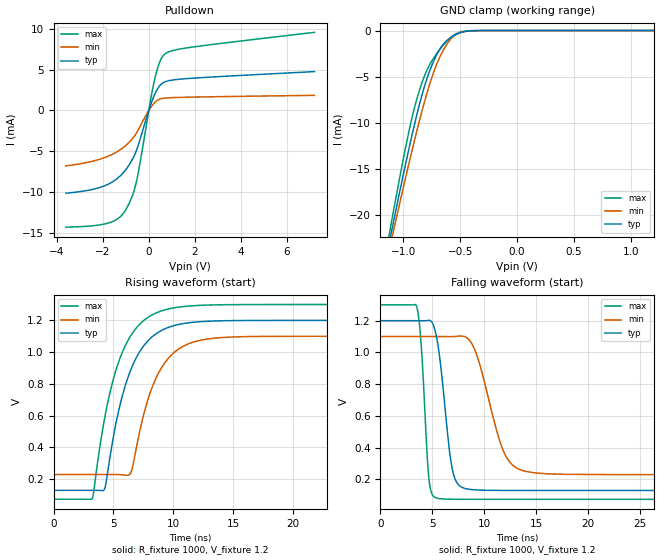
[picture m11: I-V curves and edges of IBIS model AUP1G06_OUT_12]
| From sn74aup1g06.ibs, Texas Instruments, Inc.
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[Model]   AUP1G06_OUT_12
Model_type  Open_drain
Enable   Active-Low
Vref =   1.2
Rref =   1E6
Cref =   30p
Vmeas =   0.6
| variable   typ   min   max
C_comp   1.72pF   1.50pF   1.95pF
| C_pulldown   2.12pF   1.69pF   2.59pF
| C_tri-state   1.72pF   1.50pF   1.95pF
[Temperature Range]   40   100   -40
| Ambient temperature   25   85   -40
[Voltage range]   1.2   1.1   1.3
[Pullup Reference]   1.2   1.2   1.2
[POWER Clamp Reference]   1.2   1.2   1.2
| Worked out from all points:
|   slope of the pulldown table from 0 to 0.18 V, typ, clamps not added: 125 ohm
|   GND clamp passes 1 mA (typ) near -0.61 V on its own axis
|   rising waveform, R_fixture 1000, V_fixture 1.2: 20-80 % time 2.34ns typ, 2.3ns min, 2.38ns max; typ from 0.129 V to 1.2 V
|   falling waveform, R_fixture 1000, V_fixture 1.2: 20-80 % time 1.05ns typ, 2.14ns min, 612ps max; typ from 1.2 V to 0.129 V
[GND Clamp]
| AUP1G06_OUT_12
|   Voltage   I(typ)   I(min)   I(max)
-3.6V     -193.5mA   -179.7mA   -210.2mA
-1.12V    -22.9mA    -23.71mA   -21.96mA
-1.1V     -21.68mA   -22.59mA   -20.6mA
-1.08V    -20.46mA   -21.47mA   -19.24mA
-935mV    -12.04mA   -13.67mA   -10.14mA
-835mV    -6.999mA   -8.739mA   -5.664mA
-765mV    -4.303mA   -5.73mA    -3.651mA
-690mV    -2.262mA   -3.202mA   -2.243mA
-615mV    -1.069mA   -1.462mA   -1.136mA
-550mV    -509uA     -564.1uA   -463.6uA
-340mV    -5.773uA   -7.668uA   -1.491uA
1.2V      118.1pA    564.4pA    21.05pA
[Pulldown]
| AUP1G06_OUT_12
|   Voltage   I(typ)   I(min)   I(max)
-3.6V     -10.13mA   -6.792mA   -14.3mA
-1.74V    -9.004mA   -5.576mA   -13.78mA
-1.29V    -8.143mA   -4.904mA   -13.15mA
-975mV    -7.165mA   -4.229mA   -12.05mA
-710mV    -5.969mA   -3.453mA   -10.41mA
-525mV    -4.815mA   -2.713mA   -8.581mA
90mV      761.5uA    381.6uA    1.487mA
295mV     2.185mA    1.055mA    4.264mA
495mV     3.092mA    1.407mA    6.07mA
700mV     3.505mA    1.511mA    6.919mA
1.785V    3.931mA    1.63mA     7.723mA
7.2V      4.761mA    1.852mA    9.574mA
[Ramp]
| AUP1G06_OUT_12
| variable   typ   min   max
dV/dt_r   0.64/2.34E-09   0.53/2.30E-09   0.74/2.38E-09
dV/dt_f   0.64/1.06E-09   0.52/2.14E-09   0.74/6.16E-10
R_load = 1000
[Rising Waveform]
| AUP1G06_OUT_12
R_fixture =   1000
C_fixture =   0
L_fixture =   0
V_fixture =   1.2
V_fixture_min = 1.1
V_fixture_max = 1.3
|   Time   V(typ)   V(min)   V(max)
0s        129.5mV    229.3mV    73.54mV
3.255ns   129.5mV    229.3mV    79mV
4.255ns   135.7mV    229.4mV    576.5mV
5.385ns   610.6mV    229.3mV    925.2mV
6.455ns   888mV      240.5mV    1.103V
7.66ns    1.051V     642mV      1.206V
8.7ns     1.122V     857.1mV    1.251V
10.53ns   1.175V     1.023V     1.284V
13.43ns   1.196V     1.088V     1.297V
40ns      1.2V       1.1V       1.3V
[Falling Waveform]
| AUP1G06_OUT_12
R_fixture =   1000
C_fixture =   0
L_fixture =   0
V_fixture =   1.2
V_fixture_min = 1.1
V_fixture_max = 1.3
|   Time   V(typ)   V(min)   V(max)
0s        1.2V       1.1V       1.3V
3.51ns    1.2V       1.1V       1.286V
3.94ns    1.2V       1.1V       1.038V
4.65ns    1.202V     1.1V       220mV
5.295ns   1.13V      1.1V       84.43mV
6.85ns    290.9mV    1.1V       74.21mV
7.905ns   147.4mV    1.103V     73.68mV
11.86ns   129.8mV    377.1mV    73.54mV
13.42ns   129.5mV    261.5mV    73.54mV
40ns      129.5mV    229.3mV    73.54mV
